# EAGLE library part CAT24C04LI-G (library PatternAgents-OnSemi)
CMOS Serial EEPROM
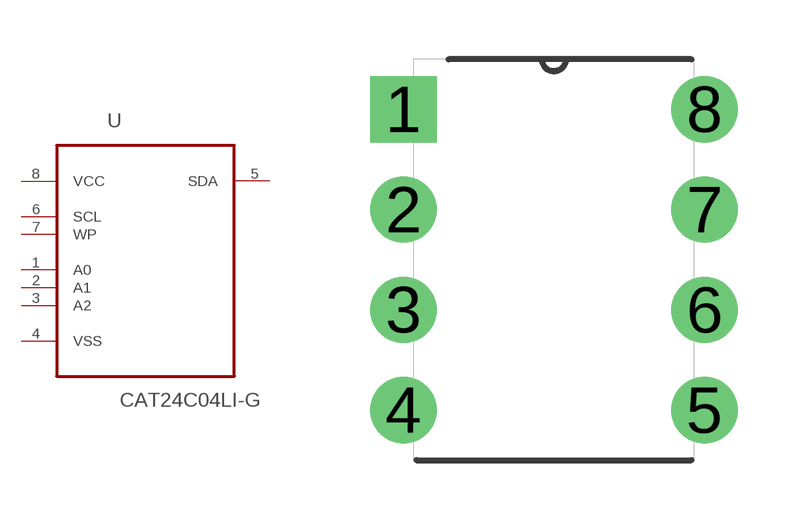
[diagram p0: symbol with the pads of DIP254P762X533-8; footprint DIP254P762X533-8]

Designator prefix U

## CAT24C04LI-G (MPN: CAT24C04LI-G; OC_FARNELL: 1718374; OC_NEWARK: 73P4460; PACKAGE: PDIP; SUPPLIER: ON SEMICONDUCTOR)  [DIP254P762X533-8]
1  A0  in
2  A1  in
3  A2  in
4  VSS  pas
5  SDA
6  SCL  in
7  WP  in
8  VCC  pwr

## Footprint DIP254P762X533-8 (pad centres in mm)
drill 1.118 square: 1 -7.62,7.62
drill 1.118: 2 -7.62,5.08; 3 -7.62,2.54; 4 -7.62,0; 5 0,0; 6 0,2.54; 7 0,5.08; 8 0,7.62

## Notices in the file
License : http://creativecommons.org/licenses/by-sa/3.0
(Creative Commons 3.0)
